|Texas Instruments Incorporated
|Low-Power, 2/8-Channel, 24-Bit Analog Front-End for Biopotential Measurements
| Marketing part#  Digital I/O Voltage Range   Package-type   #pins
|ADS1291IPBS   1.65V to 3.6 V   TQFP   32
|ADS1291IPBSR   1.65V to 3.6 V   TQFP   32
|ADS1291IRSMT   1.65V to 3.6 V   QFN   32
|ADS1291IRSMR   1.65V to 3.6 V   QFN   32
|ADS1292IPBS   1.65V to 3.6 V   TQFP   32
|ADS1292IPBSR   1.65V to 3.6 V   TQFP   32
|ADS1292RIPBS   1.65V to 3.6 V   TQFP   32
|ADS1292RIPBSR   1.65V to 3.6 V   TQFP   32
|ADS1292IRSMT   1.65V to 3.6 V   QFN   32
|ADS1292IRSMR   1.65V to 3.6 V   QFN   32
|ADS1292RIRSMT   1.65V to 3.6 V   QFN   32
|ADS1292RIRSMR   1.65V to 3.6 V   QFN   32
|ADS1294CZXGR   1.65V to 3.6 V   NFBGA   64
|ADS1294CZXGT   1.65V to 3.6 V   NFBGA   64
|ADS1294IPAG   1.65V to 3.6 V   PQFP   64
|ADS1294IPAGR   1.65V to 3.6 V   PQFP   64
|ADS1294RIZXGT   1.65V to 3.6 V   NFBGA   64
|ADS1294RIZXGR   1.65V to 3.6 V   NFBGA   64
|ADS1296CZXGR   1.65V to 3.6 V   NFBGA   64
|ADS1296CZXGT   1.65V to 3.6 V   NFBGA   64
|ADS1296IPAG   1.65V to 3.6 V   PQFP   64
|ADS1296IPAGR   1.65V to 3.6 V   PQFP   64
|ADS1296RIZXGT   1.65V to 3.6 V   NFBGA   64
|ADS1296RIZXGR   1.65V to 3.6 V   NFBGA   64
|ADS1298CZXGR   1.65V to 3.6 V   NFBGA   64
|ADS1298CZXGT   1.65V to 3.6 V   NFBGA   64
|ADS1298IPAG   1.65V to 3.6 V   PQFP   64
|ADS1298IPAGR   1.65V to 3.6 V   PQFP   64
|ADS1298RIZXGT   1.65V to 3.6 V   NFBGA   64
|ADS1298RIZXGR   1.65V to 3.6 V   NFBGA   64
|ADS1299CPAG   1.8V to 3.6 V   PQFP   64
|ADS1299CPAGR   1.8V to 3.6 V   PQFP   64
[IBIS Ver]   4.0
[File name]   ads129x.ibs
[File Rev]   1.0
[Date]   11/07/2011
[Source]   Texas Instruments Incorporated.
   Analog-eLab, HPA
   12500 TI Blvd
   Dallas, TX -75243
   For Support e-mail: elab_ibis@list.ti.com
[Notes]   Revision History:
   1.0: 01/24/2010 Initial Release
   2.0: 01/27/2010 Added ads1194/6/8 and ads1294/96
   3.0: 04/30/2010 Added marketing names for ads1294 and ads1296
   - Pin assignment based on product prelim data sheet
   ads1298.pdf
   - Initial version of the model
   - Initial Model generated from simulations in TISPICED
   - Model not matched to measurements
   - Ignore warnings related to c_comp, These are
   based on PVT variations as seen in simulations
   4.0: 11/02/2010
   - Removed references to ADS1192, ADS1196, and ADS1198 from file
   - Corrected C_comp values to true typ, min and max
   5.0: 11/18/2010
   - Added ADS1296R, ADS1294R, and ADS1294R products to this ibis
   file
   - Added ZXG R_pkg, L_pkg, and C_pkg values to the ADS1294, ADS1296,
   and ADS1298 prodcuts
   - Corrected all R_pkg, L_pkg, and C_pkg values to exclude GND and
   POWER pins from calculation
   6.0: 02/17/2011
   - Updated part numbers. The ending acronym RBZXGT is changed to RIZXGT
   and the ending acronym RBZXGR is changed to RIZXGR.
   6.1: 03/18/2011
   - Corrected part numbers to sure ADS1298R grades,
   6.2: 03/23/2011
   - Added ADS1299 products to this model.
   7.0: 04/05/2011
   - Added ADS1292 products in 32 pin TQFN package,
   8.0: 10/05/2011
   - Changed all GPIO buffers to DIO buffers. Both buffers are identical.
   - Added C_comp values that were simulated using a tank method. This
   method uses a 1nH inductor and a 1u ohm resistor.
   9.0  10/18/2011
   - Added 2.0 buffers with lagging _2 for ADS1291, ADS1292, and ADS1292R
   devices. 1.8 buffers with lagging _18 are buffers for ADS1294, ADS1296,
   and ADS1298.
   - Combined pullup data for DOUTRI_2, DIO_2, and CLK_2 is minor and
   verified with SPICE simulaton.
   10.0 11/07/2011
   - Changed voltage range for ADS1291, ADS1292, and ADS1292R. Lagging _2
   models still used with ADS1299.
   11.0 08/24/2012
   - 32 QFN package models added for ADS1291 and ADS1292
[Disclaimer]
 This product is designed as an aid for customers of Texas Instruments.
 No warranties, either expressed or implied, with respect to this third
 party software (if any) or with respect to its fitness for any
 particular purpose is claimed by Texas Instruments or the author. The
 software (if any) is provided solely on an "as is" basis. The entire
 risk as to its quality and performance is with the customer
[Copyright] (C) Copyright 2011 Texas Instruments Incorporated.
   All rights reserved.
|   ADS1299
[Component]   ads1299pag
[Manufacturer] TI
[Package]   |PAG (PQFP) - 64 pin
| variable   typ   min   max
R_pkg  0.007601   0.007601   0.007601
L_pkg  1.950031nH 1.950031nH 1.950031nH
C_pkg  0.403260pF 0.403260pF 0.403260pF
[Pin] signal_name   model_name   R_pin   L_pin   C_pin
1   IN8N   TERM   0.00802  2.18050nH  0.36893pF
2   IN8P   TERM   0.00796  2.08284nH  0.44422pF
3   IN7N   TERM   0.00774  2.00579nH  0.43874pF
4   IN7P   TERM   0.00761  1.96075nH  0.41947pF
5   IN6N   TERM   0.00767  1.93366nH  0.41193pF
6   IN6P   TERM   0.00745  1.86807nH  0.39172pF
7   IN5N   TERM   0.00723  1.80701nH  0.38069pF
8   IN5P   TERM   0.00717  1.80128nH  0.34665pF
9   IN4N   TERM   0.00717  1.80167nH  0.34655pF
10   IN4P   TERM   0.00723  1.80708nH  0.38064pF
11   IN3N   TERM   0.00746  1.86875nH  0.39156pF
12   IN3P   TERM   0.00767  1.93382nH  0.41197pF
13   IN2N   TERM   0.00762  1.96069nH  0.41976pF
14   IN2P   TERM   0.00774  2.00536nH  0.43931pF
15   IN1N   TERM   0.00796  2.08200nH  0.44472pF
16   IN1P   TERM   0.00802  2.18040nH  0.36892pF
17   TESTP_PACE_OUT1   TERM   0.00802  2.18050nH  0.36893pF
18   TESTP_PACE_OUT2   TERM   0.00796  2.08284nH  0.44422pF
19   AVDD   POWER   0.00774  2.00579nH  0.43874pF
20   AVSS   GND   0.00761  1.96075nH  0.41948pF
21   AVDD   POWER   0.00767  1.93365nH  0.41193pF
22   AVDD   POWER   0.00745  1.86807nH  0.39171pF
23   AVSS   GND   0.00723  1.80701nH  0.38069pF
24   VREFP   TERM   0.00717  1.80128nH  0.34665pF
25   VREFN   TERM   0.00717  1.80166nH  0.34656pF
26   VCAP4   TERM   0.00723  1.80707nH  0.38065pF
27   NC   NC   0.00746  1.86875nH  0.39156pF
28   VCAP1   TERM   0.00767  1.93381nH  0.41197pF
29   NC   NC   0.00762  1.96066nH  0.41979pF
30   VCAP2   TERM   0.00774  2.00511nH  0.43938pF
31   RESV1   DINPUT  0.00796  2.08195nH  0.44475pF
32   AVSS   GND   0.00802  2.18014nH  0.36899pF
33   DGND   GND   0.00802  2.18049nH  0.36893pF
34   DIN   DINPUT  0.00796  2.08283nH  0.44422pF
35   _PWDN   DINPUT  0.00774  2.00579nH  0.43874pF
36   _RESET   DINPUT  0.00761  1.96075nH  0.41947pF
37   CLK   CLK   0.00767  1.93366nH  0.41193pF
38   START   DINPUT  0.00745  1.86807nH  0.39172pF
39   _CS   DINPUT  0.00723  1.80701nH  0.38069pF
40   SCLK   DIO   0.00717  1.80128nH  0.34665pF
41   DAISY_IN   DIO   0.00717  1.80167nH  0.34655pF
42   GPIO1   DIO   0.00723  1.80708nH  0.38064pF
43   DOUT   DOUTRI  0.00746  1.86875nH  0.39156pF
44   GPIO2   DIO   0.00767  1.93382nH  0.41197pF
45   GPIO3   DIO   0.00762  1.96069nH  0.41976pF
46   GPIO4   DIO   0.00774  2.00536nH  0.43931pF
47   _DRDY   DOUTRI  0.00796  2.08200nH  0.44472pF
48   DVDD   POWER   0.00802  2.18040nH  0.36892pF
49   DGND   GND   0.00802  2.18051nH  0.36893pF
50   DVDD   POWER   0.00796  2.08284nH  0.44422pF
51   DGND   GND   0.00774  2.00579nH  0.43874pF
52   CLKSEL   DINPUT  0.00761  1.96073nH  0.41948pF
53   AVSS1   GND   0.00767  1.93366nH  0.41193pF
54   AVDD1   POWER   0.00745  1.86807nH  0.39171pF
55   VCAP3   TERM   0.00723  1.80701nH  0.38069pF
56   AVDD   POWER   0.00717  1.80128nH  0.34665pF
57   AVSS   GND   0.00717  1.80166nH  0.34656pF
58   AVSS   GND   0.00723  1.80707nH  0.38065pF
59   AVDD   POWER   0.00746  1.86875nH  0.39156pF
60   RLDREF   TERM   0.00767  1.93381nH  0.41197pF
61   RLDINV   TERM   0.00762  1.96066nH  0.41979pF
62   RLDIN   TERM   0.00774  2.00511nH  0.43938pF
63   RLDOUT   TERM   0.00796  2.08195nH  0.44475pF
64   WCT   TERM   0.00802  2.18014nH  0.36899pF
|   ADS1298
[Component]   ads1298zxg
[Manufacturer] TI
[Package]   |ZXG (PBGA) - 64 pin
| variable   typ   min   max
R_pkg  0.084959   0.084959   0.084959
L_pkg  1.726943nH 1.173300nH 2.802300nH
C_pkg  0.203317pF 0.155540pF 0.299270pF
[Pin] signal_name  model_name  R_pin  L_pin C_pin
1A   IN8P   TERM   0.080388   1.4891nH   0.16542pF
1B   IN7P   TERM   0.078742   1.4385nH   0.15797pF
1C   IN6P   TERM   0.077541   1.4231nH   0.16358pF
1D   IN5P   TERM   0.077252   1.4431nH   0.1602pF
1E   IN4P   TERM   0.076274   1.3909nH   0.16718pF
1F   IN3P   TERM   0.077401   1.4187nH   0.16692pF
1G   IN2P   TERM   0.077837   1.4526nH   0.16507pF
1H   IN1P   TERM   0.078364   1.4744nH   0.17666pF
2A   IN8N   TERM   0.078094   1.596nH   0.17296pF
2B   IN7N   TERM   0.077317   1.4768nH   0.18195pF
2C   IN6N   TERM   0.077292   1.453nH   0.17672pF
2D   IN5N   TERM   0.077416   1.4637nH   0.18795pF
2E   IN4N   TERM   0.076298   1.4016nH   0.17505pF
2F   IN3N   TERM   0.077508   1.4721nH   0.18998pF
2G   IN2N   TERM   0.077513   1.4687nH   0.18021pF
2H   IN1N   TERM   0.078587   1.5113nH   0.18073pF
3A   RLDIN   TERM   0.102240   2.3458nH   0.26608pF
3B   RLDOUT   TERM   0.086863   1.6155nH   0.20095pF
3C   RLDINV   TERM   0.098035   1.9627nH   0.23315pF
3D   WCT   TERM   0.078064   1.3941nH   0.17929pF
3E   TESTP_PACE_OUT1  TERM   0.114980   2.3577nH   0.25137pF
3F   TESTP_PACE_OUT2  TERM   0.101990   1.9882nH   0.23409pF
3G   VCAP4   TERM   0.091413   2.2569nH   0.21474pF
3H   VREFP   TERM   0.080602   1.5178nH   0.1901pF
4A   AVDD   POWER   0.044670   1.3107nH   0.45357pF
4B   AVDD   POWER   0.048649   1.5792nH   1.8442pF
4C   RLDREF   TERM   0.103750   1.931nH   0.22469pF
4D   AVSS   GND   0.014600   0.597nH   1.24pF
4E   RESV1   DINPUT   0.114160   2.8023nH   0.29927pF
4F   RESV2   TERM   0.085973   1.7256nH   0.21186pF
4G   RESV3   TERM   0.112330   2.1892nH   0.26167pF
4H   VREFN   TERM   0.071212   1.1733nH   0.16553pF
5A   AVSS   GND   0.015100   0.507nH   1.05pF
5B   AVSS   GND   0.014500   0.525nH   1.09pF
5C   AVSS   GND   0.014600   0.51nH   1.06pF
5D   AVSS   GND   0.015500   0.565nH   1.17pF
5E   GPIO4   DIO   0.106300   2.5339nH   0.28001pF
5F   GPIO1   DIO   0.103490   2.3545nH   0.28012pF
5G   _PWDN   DINPUT   0.097505   2.4515nH   0.26295pF
5H   VCAP1   TERM   0.079667   1.5368nH   0.19309pF
6A   AVDD   POWER   0.075279   1.207nH   0.57044pF
6B   AVDD   POWER   0.092725   2.1302nH   1.3472pF
6C   AVDD   POWER   0.084386   2.0005nH   1.1222pF
6D   _DRDY   DOUTRI   0.091680   2.019nH   0.23826pF
6E   GPIO3   DIO   0.092806   2.0233nH   0.22887pF
6F   DAISY_IN  DIO   0.088617   1.947nH   0.2188pF
6G   _RESET   DINPUT   0.086990   1.8608nH   0.22873pF
6H   VCAP2   TERM   0.071069   1.1744nH   0.15554pF
7A   AVDD1   POWER   0.077645   1.5948nH   0.30025pF
7B   VCAP3   TERM   0.051511   1.7265nH   0.2824pF
7C   DGND   GND   0.081013   1.9004nH   2.5639pF
7D   DGND   GND   0.054453   2.6508nH   1.2779pF
7E   GPIO2   DIO   0.079229   1.5455nH   0.20485pF
7F   _CS   DINPUT   0.076401   1.4359nH   0.20602pF
7G   START   DINPUT   0.078608   1.6115nH   0.19124pF
7H   DGND   GND   0.081108   1.8108nH   0.15779pF
8A   AVSS1   GND   0.044297   1.8219nH   0.26788pF
8B   CLKSEL   DINPUT   0.098048   2.1296nH   0.20021pF
8C   DVDD   POWER   0.073395   1.2676nH   0.87513pF
8D   DVDD   POWER   0.043758   1.9585nH   1.3668pF
8E   DOUT   DOUTRI   0.074125   1.4171nH   0.18957pF
8F   SCLK   DIO   0.073385   1.4896nH   0.17876pF
8G   CLK   CLK   0.073365   1.5643nH   0.15694pF
8H   DIN   DINPUT   0.084824   1.7114nH   0.1582pF
[Component]   ads1298pag
[Manufacturer] TI
[Package]   |PAG (PQFP) - 64 pin
| variable   typ   min   max
R_pkg  0.007601   0.007601   0.007601
L_pkg  1.950031nH 1.950031nH 1.950031nH
C_pkg  0.403260pF 0.403260pF 0.403260pF
[Pin] signal_name   model_name   R_pin   L_pin   C_pin
1   IN8N   TERM   0.00802  2.18050nH  0.36893pF
2   IN8P   TERM   0.00796  2.08284nH  0.44422pF
3   IN7N   TERM   0.00774  2.00579nH  0.43874pF
4   IN7P   TERM   0.00761  1.96075nH  0.41947pF
5   IN6N   TERM   0.00767  1.93366nH  0.41193pF
6   IN6P   TERM   0.00745  1.86807nH  0.39172pF
7   IN5N   TERM   0.00723  1.80701nH  0.38069pF
8   IN5P   TERM   0.00717  1.80128nH  0.34665pF
9   IN4N   TERM   0.00717  1.80167nH  0.34655pF
10   IN4P   TERM   0.00723  1.80708nH  0.38064pF
11   IN3N   TERM   0.00746  1.86875nH  0.39156pF
12   IN3P   TERM   0.00767  1.93382nH  0.41197pF
13   IN2N   TERM   0.00762  1.96069nH  0.41976pF
14   IN2P   TERM   0.00774  2.00536nH  0.43931pF
15   IN1N   TERM   0.00796  2.08200nH  0.44472pF
16   IN1P   TERM   0.00802  2.18040nH  0.36892pF
17   TESTP_PACE_OUT1   TERM   0.00802  2.18050nH  0.36893pF
18   TESTP_PACE_OUT2   TERM   0.00796  2.08284nH  0.44422pF
19   AVDD   POWER   0.00774  2.00579nH  0.43874pF
20   AVSS   GND   0.00761  1.96075nH  0.41948pF
21   AVDD   POWER   0.00767  1.93365nH  0.41193pF
22   AVDD   POWER   0.00745  1.86807nH  0.39171pF
23   AVSS   GND   0.00723  1.80701nH  0.38069pF
24   VREFP   TERM   0.00717  1.80128nH  0.34665pF
25   VREFN   TERM   0.00717  1.80166nH  0.34656pF
26   VCAP4   TERM   0.00723  1.80707nH  0.38065pF
27   NC   NC   0.00746  1.86875nH  0.39156pF
28   VCAP1   TERM   0.00767  1.93381nH  0.41197pF
29   NC   NC   0.00762  1.96066nH  0.41979pF
30   VCAP2   TERM   0.00774  2.00511nH  0.43938pF
31   RESV1   DINPUT  0.00796  2.08195nH  0.44475pF
32   AVSS   GND   0.00802  2.18014nH  0.36899pF
33   DGND   GND   0.00802  2.18049nH  0.36893pF
34   DIN   DINPUT  0.00796  2.08283nH  0.44422pF
35   _PWDN   DINPUT  0.00774  2.00579nH  0.43874pF
36   _RESET   DINPUT  0.00761  1.96075nH  0.41947pF
37   CLK   CLK   0.00767  1.93366nH  0.41193pF
38   START   DINPUT  0.00745  1.86807nH  0.39172pF
39   _CS   DINPUT  0.00723  1.80701nH  0.38069pF
40   SCLK   DIO   0.00717  1.80128nH  0.34665pF
41   DAISY_IN   DIO   0.00717  1.80167nH  0.34655pF
42   GPIO1   DIO   0.00723  1.80708nH  0.38064pF
43   DOUT   DOUTRI  0.00746  1.86875nH  0.39156pF
44   GPIO2   DIO   0.00767  1.93382nH  0.41197pF
45   GPIO3   DIO   0.00762  1.96069nH  0.41976pF
46   GPIO4   DIO   0.00774  2.00536nH  0.43931pF
47   _DRDY   DOUTRI  0.00796  2.08200nH  0.44472pF
48   DVDD   POWER   0.00802  2.18040nH  0.36892pF
49   DGND   GND   0.00802  2.18051nH  0.36893pF
50   DVDD   POWER   0.00796  2.08284nH  0.44422pF
51   DGND   GND   0.00774  2.00579nH  0.43874pF
52   CLKSEL   DINPUT  0.00761  1.96073nH  0.41948pF
53   AVSS1   GND   0.00767  1.93366nH  0.41193pF
54   AVDD1   POWER   0.00745  1.86807nH  0.39171pF
55   VCAP3   TERM   0.00723  1.80701nH  0.38069pF
56   AVDD   POWER   0.00717  1.80128nH  0.34665pF
57   AVSS   GND   0.00717  1.80166nH  0.34656pF
58   AVSS   GND   0.00723  1.80707nH  0.38065pF
59   AVDD   POWER   0.00746  1.86875nH  0.39156pF
60   RLDREF   TERM   0.00767  1.93381nH  0.41197pF
61   RLDINV   TERM   0.00762  1.96066nH  0.41979pF
62   RLDIN   TERM   0.00774  2.00511nH  0.43938pF
63   RLDOUT   TERM   0.00796  2.08195nH  0.44475pF
64   WCT   TERM   0.00802  2.18014nH  0.36899pF
|   ADS1296
[Component]   ads1296zxg
[Manufacturer] TI
[Package]   |ZXG (PBGA) - 64 pin
| variable   typ   min   max
R_pkg  0.084959   0.084959   0.084959
L_pkg  1.726943nH 1.173300nH 2.802300nH
C_pkg  0.203317pF 0.155540pF 0.299270pF
[Pin] signal_name  model_name  R_pin  L_pin C_pin
1A   NC   NC   0.080388   1.4891nH   0.16542pF
1B   NC   NC   0.078742   1.4385nH   0.15797pF
1C   IN6P   TERM   0.077541   1.4231nH   0.16358pF
1D   IN5P   TERM   0.077252   1.4431nH   0.1602pF
1E   IN4P   TERM   0.076274   1.3909nH   0.16718pF
1F   IN3P   TERM   0.077401   1.4187nH   0.16692pF
1G   IN2P   TERM   0.077837   1.4526nH   0.16507pF
1H   IN1P   TERM   0.078364   1.4744nH   0.17666pF
2A   NC   NC   0.078094   1.596nH   0.17296pF
2B   NC   NC   0.077317   1.4768nH   0.18195pF
2C   IN6N   TERM   0.077292   1.453nH   0.17672pF
2D   IN5N   TERM   0.077416   1.4637nH   0.18795pF
2E   IN4N   TERM   0.076298   1.4016nH   0.17505pF
2F   IN3N   TERM   0.077508   1.4721nH   0.18998pF
2G   IN2N   TERM   0.077513   1.4687nH   0.18021pF
2H   IN1N   TERM   0.078587   1.5113nH   0.18073pF
3A   RLDIN   TERM   0.102240   2.3458nH   0.26608pF
3B   RLDOUT   TERM   0.086863   1.6155nH   0.20095pF
3C   RLDINV   TERM   0.098035   1.9627nH   0.23315pF
3D   WCT   TERM   0.078064   1.3941nH   0.17929pF
3E   TESTP_PACE_OUT1  TERM   0.114980   2.3577nH   0.25137pF
3F   TESTP_PACE_OUT2  TERM   0.101990   1.9882nH   0.23409pF
3G   VCAP4   TERM   0.091413   2.2569nH   0.21474pF
3H   VREFP   TERM   0.080602   1.5178nH   0.1901pF
4A   AVDD   POWER   0.044670   1.3107nH   0.45357pF
4B   AVDD   POWER   0.048649   1.5792nH   1.8442pF
4C   RLDREF   TERM   0.103750   1.931nH   0.22469pF
4D   AVSS   GND   0.014600   0.597nH   1.24pF
4E   RESV1   DINPUT   0.114160   2.8023nH   0.29927pF
4F   RESV2   TERM   0.085973   1.7256nH   0.21186pF
4G   RESV3   TERM   0.112330   2.1892nH   0.26167pF
4H   VREFN   TERM   0.071212   1.1733nH   0.16553pF
5A   AVSS   GND   0.015100   0.507nH   1.05pF
5B   AVSS   GND   0.014500   0.525nH   1.09pF
5C   AVSS   GND   0.014600   0.51nH   1.06pF
5D   AVSS   GND   0.015500   0.565nH   1.17pF
5E   GPIO4   DIO   0.106300   2.5339nH   0.28001pF
5F   GPIO1   DIO   0.103490   2.3545nH   0.28012pF
5G   _PWDN   DINPUT   0.097505   2.4515nH   0.26295pF
5H   VCAP1   TERM   0.079667   1.5368nH   0.19309pF
6A   AVDD   POWER   0.075279   1.207nH   0.57044pF
6B   AVDD   POWER   0.092725   2.1302nH   1.3472pF
6C   AVDD   POWER   0.084386   2.0005nH   1.1222pF
6D   _DRDY   DOUTRI   0.091680   2.019nH   0.23826pF
6E   GPIO3   DIO   0.092806   2.0233nH   0.22887pF
6F   DAISY_IN  DIO   0.088617   1.947nH   0.2188pF
6G   _RESET   DINPUT   0.086990   1.8608nH   0.22873pF
6H   VCAP2   TERM   0.071069   1.1744nH   0.15554pF
7A   AVDD1   POWER   0.077645   1.5948nH   0.30025pF
7B   VCAP3   TERM   0.051511   1.7265nH   0.2824pF
7C   DGND   GND   0.081013   1.9004nH   2.5639pF
7D   DGND   GND   0.054453   2.6508nH   1.2779pF
7E   GPIO2   DIO   0.079229   1.5455nH   0.20485pF
7F   _CS   DINPUT   0.076401   1.4359nH   0.20602pF
7G   START   DINPUT   0.078608   1.6115nH   0.19124pF
7H   DGND   GND   0.081108   1.8108nH   0.15779pF
8A   AVSS1   GND   0.044297   1.8219nH   0.26788pF
8B   CLKSEL   DINPUT   0.098048   2.1296nH   0.20021pF
8C   DVDD   POWER   0.073395   1.2676nH   0.87513pF
8D   DVDD   POWER   0.043758   1.9585nH   1.3668pF
8E   DOUT   DOUTRI   0.074125   1.4171nH   0.18957pF
8F   SCLK   DIO   0.073385   1.4896nH   0.17876pF
8G   CLK   CLK   0.073365   1.5643nH   0.15694pF
8H   DIN   DINPUT   0.084824   1.7114nH   0.1582pF
[Component]   ads1296pag
[Manufacturer] TI
[Package]   |PAG (PQFP) - 64 pin
| variable   typ   min   max
R_pkg  0.007601   0.007601   0.007601
L_pkg  1.950031nH 1.950031nH 1.950031nH
C_pkg  0.403260pF 0.403260pF 0.403260pF
[Pin] signal_name   model_name   R_pin   L_pin   C_pin
1   NC   NC   0.00802  2.18050nH  0.36893pF
2   NC   NC   0.00796  2.08284nH  0.44422pF
3   NC   NC   0.00774  2.00579nH  0.43874pF
4   NC   NC   0.00761  1.96075nH  0.41947pF
5   IN6N   TERM   0.00767  1.93366nH  0.41193pF
6   IN6P   TERM   0.00745  1.86807nH  0.39172pF
7   IN5N   TERM   0.00723  1.80701nH  0.38069pF
8   IN5P   TERM   0.00717  1.80128nH  0.34665pF
9   IN4N   TERM   0.00717  1.80167nH  0.34655pF
10   IN4P   TERM   0.00723  1.80708nH  0.38064pF
11   IN3N   TERM   0.00746  1.86875nH  0.39156pF
12   IN3P   TERM   0.00767  1.93382nH  0.41197pF
13   IN2N   TERM   0.00762  1.96069nH  0.41976pF
14   IN2P   TERM   0.00774  2.00536nH  0.43931pF
15   IN1N   TERM   0.00796  2.08200nH  0.44472pF
16   IN1P   TERM   0.00802  2.18040nH  0.36892pF
17   TESTP_PACE_OUT1   TERM   0.00802  2.18050nH  0.36893pF
18   TESTP_PACE_OUT2   TERM   0.00796  2.08284nH  0.44422pF
19   AVDD   POWER   0.00774  2.00579nH  0.43874pF
20   AVSS   GND   0.00761  1.96075nH  0.41948pF
21   AVDD   POWER   0.00767  1.93365nH  0.41193pF
22   AVDD   POWER   0.00745  1.86807nH  0.39171pF
23   AVSS   GND   0.00723  1.80701nH  0.38069pF
24   VREFP   TERM   0.00717  1.80128nH  0.34665pF
25   VREFN   TERM   0.00717  1.80166nH  0.34656pF
26   VCAP4   TERM   0.00723  1.80707nH  0.38065pF
27   NC   NC   0.00746  1.86875nH  0.39156pF
28   VCAP1   TERM   0.00767  1.93381nH  0.41197pF
29   NC   NC   0.00762  1.96066nH  0.41979pF
30   VCAP2   TERM   0.00774  2.00511nH  0.43938pF
31   RESV1   DINPUT  0.00796  2.08195nH  0.44475pF
32   AVSS   GND   0.00802  2.18014nH  0.36899pF
33   DGND   GND   0.00802  2.18049nH  0.36893pF
34   DIN   DINPUT  0.00796  2.08283nH  0.44422pF
35   _PWDN   DINPUT  0.00774  2.00579nH  0.43874pF
36   _RESET   DINPUT  0.00761  1.96075nH  0.41947pF
37   CLK   CLK   0.00767  1.93366nH  0.41193pF
38   START   DINPUT  0.00745  1.86807nH  0.39172pF
39   _CS   DINPUT  0.00723  1.80701nH  0.38069pF
40   SCLK   DIO   0.00717  1.80128nH  0.34665pF
41   DAISY_IN   DIO   0.00717  1.80167nH  0.34655pF
42   GPIO1   DIO   0.00723  1.80708nH  0.38064pF
43   DOUT   DOUTRI  0.00746  1.86875nH  0.39156pF
44   GPIO2   DIO   0.00767  1.93382nH  0.41197pF
45   GPIO3   DIO   0.00762  1.96069nH  0.41976pF
46   GPIO4   DIO   0.00774  2.00536nH  0.43931pF
47   _DRDY   DOUTRI  0.00796  2.08200nH  0.44472pF
48   DVDD   POWER   0.00802  2.18040nH  0.36892pF
49   DGND   GND   0.00802  2.18051nH  0.36893pF
50   DVDD   POWER   0.00796  2.08284nH  0.44422pF
51   DGND   GND   0.00774  2.00579nH  0.43874pF
52   CLKSEL   DINPUT  0.00761  1.96073nH  0.41948pF
53   AVSS1   GND   0.00767  1.93366nH  0.41193pF
54   AVDD1   POWER   0.00745  1.86807nH  0.39171pF
55   VCAP3   TERM   0.00723  1.80701nH  0.38069pF
56   AVDD   POWER   0.00717  1.80128nH  0.34665pF
57   AVSS   GND   0.00717  1.80166nH  0.34656pF
58   AVSS   GND   0.00723  1.80707nH  0.38065pF
59   AVDD   POWER   0.00746  1.86875nH  0.39156pF
60   RLDREF   TERM   0.00767  1.93381nH  0.41197pF
61   RLDINV   TERM   0.00762  1.96066nH  0.41979pF
62   RLDIN   TERM   0.00774  2.00511nH  0.43938pF
63   RLDOUT   TERM   0.00796  2.08195nH  0.44475pF
64   WCT   TERM   0.00802  2.18014nH  0.36899pF
|   ADS1294
[Component]   ads1294zxg
[Manufacturer] TI
[Package]   |ZXG (PBGA) - 64 pin
| variable   typ   min   max
R_pkg  0.084959   0.084959   0.084959
L_pkg  1.726943nH 1.173300nH 2.802300nH
C_pkg  0.203317pF 0.155540pF 0.299270pF
[Pin] signal_name  model_name  R_pin  L_pin C_pin
1A   NC   NC   0.080388   1.4891nH   0.16542pF
1B   NC   NC   0.078742   1.4385nH   0.15797pF
1C   NC   NC   0.077541   1.4231nH   0.16358pF
1D   NC   NC   0.077252   1.4431nH   0.1602pF
1E   IN4P   TERM   0.076274   1.3909nH   0.16718pF
1F   IN3P   TERM   0.077401   1.4187nH   0.16692pF
1G   IN2P   TERM   0.077837   1.4526nH   0.16507pF
1H   IN1P   TERM   0.078364   1.4744nH   0.17666pF
2A   NC   NC   0.078094   1.596nH   0.17296pF
2B   NC   NC   0.077317   1.4768nH   0.18195pF
2C   NC   NC   0.077292   1.453nH   0.17672pF
2D   NC   NC   0.077416   1.4637nH   0.18795pF
2E   IN4N   TERM   0.076298   1.4016nH   0.17505pF
2F   IN3N   TERM   0.077508   1.4721nH   0.18998pF
2G   IN2N   TERM   0.077513   1.4687nH   0.18021pF
2H   IN1N   TERM   0.078587   1.5113nH   0.18073pF
3A   RLDIN   TERM   0.102240   2.3458nH   0.26608pF
3B   RLDOUT   TERM   0.086863   1.6155nH   0.20095pF
3C   RLDINV   TERM   0.098035   1.9627nH   0.23315pF
3D   WCT   TERM   0.078064   1.3941nH   0.17929pF
3E   TESTP_PACE_OUT1  TERM   0.114980   2.3577nH   0.25137pF
3F   TESTP_PACE_OUT2  TERM   0.101990   1.9882nH   0.23409pF
3G   VCAP4   TERM   0.091413   2.2569nH   0.21474pF
3H   VREFP   TERM   0.080602   1.5178nH   0.1901pF
4A   AVDD   POWER   0.044670   1.3107nH   0.45357pF
4B   AVDD   POWER   0.048649   1.5792nH   1.8442pF
4C   RLDREF   TERM   0.103750   1.931nH   0.22469pF
4D   AVSS   GND   0.014600   0.597nH   1.24pF
4E   RESV1   DINPUT   0.114160   2.8023nH   0.29927pF
4F   RESV2   TERM   0.085973   1.7256nH   0.21186pF
4G   RESV3   TERM   0.112330   2.1892nH   0.26167pF
4H   VREFN   TERM   0.071212   1.1733nH   0.16553pF
5A   AVSS   GND   0.015100   0.507nH   1.05pF
5B   AVSS   GND   0.014500   0.525nH   1.09pF
5C   AVSS   GND   0.014600   0.51nH   1.06pF
5D   AVSS   GND   0.015500   0.565nH   1.17pF
5E   GPIO4   DIO   0.106300   2.5339nH   0.28001pF
5F   GPIO1   DIO   0.103490   2.3545nH   0.28012pF
5G   _PWDN   DINPUT   0.097505   2.4515nH   0.26295pF
5H   VCAP1   TERM   0.079667   1.5368nH   0.19309pF
6A   AVDD   POWER   0.075279   1.207nH   0.57044pF
6B   AVDD   POWER   0.092725   2.1302nH   1.3472pF
6C   AVDD   POWER   0.084386   2.0005nH   1.1222pF
6D   _DRDY   DOUTRI   0.091680   2.019nH   0.23826pF
6E   GPIO3   DIO   0.092806   2.0233nH   0.22887pF
6F   DAISY_IN  DIO   0.088617   1.947nH   0.2188pF
6G   _RESET   DINPUT   0.086990   1.8608nH   0.22873pF
6H   VCAP2   TERM   0.071069   1.1744nH   0.15554pF
7A   AVDD1   POWER   0.077645   1.5948nH   0.30025pF
7B   VCAP3   TERM   0.051511   1.7265nH   0.2824pF
7C   DGND   GND   0.081013   1.9004nH   2.5639pF
7D   DGND   GND   0.054453   2.6508nH   1.2779pF
7E   GPIO2   DIO   0.079229   1.5455nH   0.20485pF
7F   _CS   DINPUT   0.076401   1.4359nH   0.20602pF
7G   START   DINPUT   0.078608   1.6115nH   0.19124pF
7H   DGND   GND   0.081108   1.8108nH   0.15779pF
8A   AVSS1   GND   0.044297   1.8219nH   0.26788pF
8B   CLKSEL   DINPUT   0.098048   2.1296nH   0.20021pF
8C   DVDD   POWER   0.073395   1.2676nH   0.87513pF
8D   DVDD   POWER   0.043758   1.9585nH   1.3668pF
8E   DOUT   DOUTRI   0.074125   1.4171nH   0.18957pF
8F   SCLK   DIO   0.073385   1.4896nH   0.17876pF
8G   CLK   CLK   0.073365   1.5643nH   0.15694pF
8H   DIN   DINPUT   0.084824   1.7114nH   0.1582pF
[Component]   ads1294pag
[Manufacturer] TI
[Package]   |PAG (PQFP) - 64 pin
| variable   typ   min   max
R_pkg  0.007601   0.007601   0.007601
L_pkg  1.950031nH 1.950031nH 1.950031nH
C_pkg  0.403260pF 0.403260pF 0.403260pF
[Pin] signal_name   model_name   R_pin   L_pin   C_pin
1   IN8N   NC   0.00802  2.18050nH  0.36893pF
2   IN8P   NC   0.00796  2.08284nH  0.44422pF
3   IN7N   NC   0.00774  2.00579nH  0.43874pF
4   IN7P   NC   0.00761  1.96075nH  0.41947pF
5   IN6N   NC   0.00767  1.93366nH  0.41193pF
6   IN6P   NC   0.00745  1.86807nH  0.39172pF
7   IN5N   NC   0.00723  1.80701nH  0.38069pF
8   IN5P   NC   0.00717  1.80128nH  0.34665pF
9   IN4N   TERM   0.00717  1.80167nH  0.34655pF
10   IN4P   TERM   0.00723  1.80708nH  0.38064pF
11   IN3N   TERM   0.00746  1.86875nH  0.39156pF
12   IN3P   TERM   0.00767  1.93382nH  0.41197pF
13   IN2N   TERM   0.00762  1.96069nH  0.41976pF
14   IN2P   TERM   0.00774  2.00536nH  0.43931pF
15   IN1N   TERM   0.00796  2.08200nH  0.44472pF
16   IN1P   TERM   0.00802  2.18040nH  0.36892pF
17   TESTP_PACE_OUT1   TERM   0.00802  2.18050nH  0.36893pF
18   TESTP_PACE_OUT2   TERM   0.00796  2.08284nH  0.44422pF
19   AVDD   POWER   0.00774  2.00579nH  0.43874pF
20   AVSS   GND   0.00761  1.96075nH  0.41948pF
21   AVDD   POWER   0.00767  1.93365nH  0.41193pF
22   AVDD   POWER   0.00745  1.86807nH  0.39171pF
23   AVSS   GND   0.00723  1.80701nH  0.38069pF
24   VREFP   TERM   0.00717  1.80128nH  0.34665pF
25   VREFN   TERM   0.00717  1.80166nH  0.34656pF
26   VCAP4   TERM   0.00723  1.80707nH  0.38065pF
27   NC   NC   0.00746  1.86875nH  0.39156pF
28   VCAP1   TERM   0.00767  1.93381nH  0.41197pF
29   NC   NC   0.00762  1.96066nH  0.41979pF
30   VCAP2   TERM   0.00774  2.00511nH  0.43938pF
31   RESV1   DINPUT  0.00796  2.08195nH  0.44475pF
32   AVSS   GND   0.00802  2.18014nH  0.36899pF
33   DGND   GND   0.00802  2.18049nH  0.36893pF
34   DIN   DINPUT  0.00796  2.08283nH  0.44422pF
35   _PWDN   DINPUT  0.00774  2.00579nH  0.43874pF
36   _RESET   DINPUT  0.00761  1.96075nH  0.41947pF
37   CLK   CLK   0.00767  1.93366nH  0.41193pF
38   START   DINPUT  0.00745  1.86807nH  0.39172pF
39   _CS   DINPUT  0.00723  1.80701nH  0.38069pF
40   SCLK   DIO   0.00717  1.80128nH  0.34665pF
41   DAISY_IN   DIO   0.00717  1.80167nH  0.34655pF
42   GPIO1   DIO   0.00723  1.80708nH  0.38064pF
43   DOUT   DOUTRI  0.00746  1.86875nH  0.39156pF
44   GPIO2   DIO   0.00767  1.93382nH  0.41197pF
45   GPIO3   DIO   0.00762  1.96069nH  0.41976pF
46   GPIO4   DIO   0.00774  2.00536nH  0.43931pF
47   _DRDY   DOUTRI  0.00796  2.08200nH  0.44472pF
48   DVDD   POWER   0.00802  2.18040nH  0.36892pF
49   DGND   GND   0.00802  2.18051nH  0.36893pF
50   DVDD   POWER   0.00796  2.08284nH  0.44422pF
51   DGND   GND   0.00774  2.00579nH  0.43874pF
52   CLKSEL   DINPUT  0.00761  1.96073nH  0.41948pF
53   AVSS1   GND   0.00767  1.93366nH  0.41193pF
54   AVDD1   POWER   0.00745  1.86807nH  0.39171pF
55   VCAP3   TERM   0.00723  1.80701nH  0.38069pF
56   AVDD   POWER   0.00717  1.80128nH  0.34665pF
57   AVSS   GND   0.00717  1.80166nH  0.34656pF
58   AVSS   GND   0.00723  1.80707nH  0.38065pF
59   AVDD   POWER   0.00746  1.86875nH  0.39156pF
60   RLDREF   TERM   0.00767  1.93381nH  0.41197pF
61   RLDINV   TERM   0.00762  1.96066nH  0.41979pF
62   RLDIN   TERM   0.00774  2.00511nH  0.43938pF
63   RLDOUT   TERM   0.00796  2.08195nH  0.44475pF
64   WCT   TERM   0.00802  2.18014nH  0.36899pF
|   ADS1292
[Component]   ads1292pbs
[Manufacturer] TI
[Package]   |PBS (TQFP) - 32 pin
| variable   typ   min   max
R_pkg   5.66263E-02   3.17700E-02   6.22300E-02
L_pkg   1.90859E+00nH 1.58036E+00nH 2.05660E+00nH
C_pkg   3.94649E-01pF 3.77910E-01pF 4.24640E-01pF
[Pin] signal_name   model_name   R_pin   L_pin   C_pin
1   PGA1N   TERM   0.06036  2.03101nH  0.37977pF
2   PGA1P   TERM   0.05911  1.95272nH  0.41005pF
3   IN1N   TERM   0.05831  1.88394nH  0.39201pF
4   IN1P   TERM   0.05810  1.84984nH  0.38129pF
5   IN2N   TERM   0.05810  1.85071nH  0.38135pF
6   IN2P   TERM   0.05832  1.88654nH  0.39223pF
7   PGA2N   TERM   0.05914  1.95753nH  0.41031pF
8   PGA2P   TERM   0.06041  2.03829nH  0.37970pF
9   VREFP   TERM   0.06011  2.03502nH  0.38025pF
10  VREFN   TERM   0.05849  1.94859nH  0.41037pF
11  VCAP1   TERM   0.05826  1.88956nH  0.39248pF
12  GPIO1/RCLK   DIO   0.03177  1.59232nH  0.41419pF
13  GPIO2/RCLK   DIO   0.03187  1.58036nH  0.41607pF
14  CLKSEL   DINPUT 0.05892  1.90189nH  0.39388pF
15  _PWDN/_RESET   DINPUT 0.05833  1.94540nH  0.41154pF
16  START   DINPUT 0.06005  2.03312nH  0.38068pF
17  CLK   CLK   0.06132  2.05652nH  0.38073pF
18  _CS   DINPUT 0.05940  1.96335nH  0.41136pF
19  DIN   DINPUT 0.05800  1.88100nH  0.39302pF
20  SCLK   DINPUT 0.05841  1.85614nH  0.38258pF
21  DOUT   DOUTRI 0.05918  1.86987nH  0.38231pF
22  _DRDY   DIO   0.05941  1.90531nH  0.39279pF
23  DVDD   POWER  0.06108  1.99071nH  0.41314pF
24  DGND   GND   0.06520  2.12375nH  0.38560pF
25  GPIO2/RCLK2   DIO   0.05982  2.02375nH  0.37791pF
26  GPIO1/RCLK1   DIO   0.05924  1.95629nH  0.40891pF
27  VCAP2   TERM   0.03343  1.67142nH  0.42464pF
28  RLDINV   TERM   0.06223  1.92683nH  0.38751pF
29  RLDIN/RLDREF   TERM   0.05963  1.87740nH  0.38482pF
30  RLDOUT   TERM   0.05832  1.88335nH  0.39358pF
31  RESP_MODP/IN3P TERM   0.05911  1.95300nH  0.41148pF
32  RESP_MODN/IN3N TERM   0.06164  2.05660nH  0.38167pF
|   ADS1292
[Component]   ads1292rsm
[Manufacturer] TI
[Package]   |RSM (QFN) - 32 pin
| variable   typ   min   max
R_pkg   0.0644   0.0330   0.0768
L_pkg   0.8006nH 0.5037nH 0.9598nH
C_pkg   0.1360pF 0.1213pF 0.1671pF
[Pin] signal_name   model_name   R_pin   L_pin   C_pin
1   PGA1N   TERM   0.06981   0.86398nH   0.12266pF
2   PGA1P   TERM   0.06734   0.82828nH   0.13736pF
3   IN1N   TERM   0.06549   0.80232nH   0.13536pF
4   IN1P   TERM   0.06467   0.7907nH   0.13341pF
5   IN2N   TERM   0.06467   0.7907nH   0.13342pF
6   IN2P   TERM   0.06549   0.80234nH   0.13537pF
7   PGA2N   TERM   0.06734   0.82831nH   0.1374pF
8   PGA2P   TERM   0.06982   0.86408nH   0.12324pF
9   VREFP   TERM   0.06941   0.85736nH   0.12314pF
10   VREFN   TERM   0.06537   0.79827nH   0.13606pF
11   VCAP1   TERM   0.06447   0.78457nH   0.1347pF
12   GPIO1/RCLK   DIO   0.03298   0.51461nH   0.1614pF
13   GPIO2/RCLK   DIO   0.03311   0.50367nH   0.16305pF
14   CLKSEL   DINPUT   0.06526   0.79658nH   0.13595pF
15   _PWDN/_RESET   DINPUT   0.06504   0.79185nH   0.13645pF
16   START   DINPUT   0.0693   0.85128nH   0.12337pF
17   CLK   CLK   0.07116   0.87727nH   0.1242pF
18   _CS   DINPUT   0.06777   0.82756nH   0.13844pF
19   DIN   DINPUT   0.06481   0.78556nH   0.13548pF
20   SCLK   DINPUT   0.06507   0.78889nH   0.13429pF
21   DOUT   DOUTRI   0.06646   0.80858nH   0.13514pF
22   _DRDY   DIO   0.0674   0.82218nH   0.13734pF
23   DVDD   POWER   0.07055   0.86775nH   0.14182pF
24   DGND   GND   0.07677   0.95983nH   0.13053pF
25   GPIO2/RCLK2   DIO   0.0689   0.84568nH   0.1213pF
26   GPIO1/RCLK1   DIO   0.06673   0.81477nH   0.13627pF
27   VCAP2   TERM   0.03588   0.58479nH   0.16713pF
28   RLDINV   TERM   0.07055   0.86802nH   0.14129pF
29   RLDIN/RLDREF   TERM   0.06633   0.80886nH   0.13681pF
30   RLDOUT   TERM   0.06454   0.78561nH   0.13566pF
31   RESP_MODP/IN3P   TERM   0.06653   0.81501nH   0.13796pF
32   RESP_MODN/IN3N   TERM   0.07165   0.89005nH   0.12572pF
|   ADS1291
[Component]   ads1291pbs
[Manufacturer] TI
[Package]   |PBS (TQFP) - 32 pin
| variable   typ   min   max
R_pkg   5.66263E-02   3.17700E-02   6.22300E-02
L_pkg   1.90859E+00nH 1.58036E+00nH 2.05660E+00nH
C_pkg   3.94649E-01pF 3.77910E-01pF 4.24640E-01pF
[Pin] signal_name   model_name   R_pin   L_pin   C_pin
1   PGA1N   TERM   0.06036  2.03101nH  0.37977pF
2   PGA1P   TERM   0.05911  1.95272nH  0.41005pF
3   IN1N   TERM   0.05831  1.88394nH  0.39201pF
4   IN1P   TERM   0.05810  1.84984nH  0.38129pF
5   IN2N   TERM   0.05810  1.85071nH  0.38135pF
6   IN2P   TERM   0.05832  1.88654nH  0.39223pF
7   PGA2N   TERM   0.05914  1.95753nH  0.41031pF
8   PGA2P   TERM   0.06041  2.03829nH  0.37970pF
9   VREFP   TERM   0.06011  2.03502nH  0.38025pF
10  VREFN   TERM   0.05849  1.94859nH  0.41037pF
11  VCAP1   TERM   0.05826  1.88956nH  0.39248pF
12  GPIO1/RCLK   DIO   0.03177  1.59232nH  0.41419pF
13  GPIO2/RCLK   DIO   0.03187  1.58036nH  0.41607pF
14  CLKSEL   DINPUT 0.05892  1.90189nH  0.39388pF
15  _PWDN/_RESET   DINPUT 0.05833  1.94540nH  0.41154pF
16  START   DINPUT 0.06005  2.03312nH  0.38068pF
17  CLK   CLK   0.06132  2.05652nH  0.38073pF
18  _CS   DINPUT 0.05940  1.96335nH  0.41136pF
19  DIN   DINPUT 0.05800  1.88100nH  0.39302pF
20  SCLK   DINPUT 0.05841  1.85614nH  0.38258pF
21  DOUT   DOUTRI 0.05918  1.86987nH  0.38231pF
22  _DRDY   DIO   0.05941  1.90531nH  0.39279pF
23  DVDD   POWER  0.06108  1.99071nH  0.41314pF
24  DGND   GND   0.06520  2.12375nH  0.38560pF
25  NC   TERM   0.05982  2.02375nH  0.37791pF
26  NC   TERM   0.05924  1.95629nH  0.40891pF
27  VCAP2   TERM   0.03343  1.67142nH  0.42464pF
28  RLDINV   TERM   0.06223  1.92683nH  0.38751pF
29  RLDIN/RLDREF   TERM   0.05963  1.87740nH  0.38482pF
30  RLDOUT   TERM   0.05832  1.88335nH  0.39358pF
31  RESP_MODP/IN3P TERM   0.05911  1.95300nH  0.41148pF
32  RESP_MODN/IN3N TERM   0.06164  2.05660nH  0.38167pF
|   ADS1291
[Component]   ads1291rsm
[Manufacturer] TI
[Package]   |RSM (QFN) - 32 pin
| variable   typ   min   max
R_pkg   0.0644   0.0330   0.0768
L_pkg   0.8006nH 0.5037nH 0.9598nH
C_pkg   0.1360pF 0.1213pF 0.1671pF
[Pin] signal_name   model_name   R_pin   L_pin   C_pin
1   PGA1N   TERM   0.06981   0.86398nH   0.12266pF
2   PGA1P   TERM   0.06734   0.82828nH   0.13736pF
3   IN1N   TERM   0.06549   0.80232nH   0.13536pF
4   IN1P   TERM   0.06467   0.7907nH   0.13341pF
5   IN2N   TERM   0.06467   0.7907nH   0.13342pF
6   IN2P   TERM   0.06549   0.80234nH   0.13537pF
7   PGA2N   TERM   0.06734   0.82831nH   0.1374pF
8   PGA2P   TERM   0.06982   0.86408nH   0.12324pF
9   VREFP   TERM   0.06941   0.85736nH   0.12314pF
10   VREFN   TERM   0.06537   0.79827nH   0.13606pF
11   VCAP1   TERM   0.06447   0.78457nH   0.1347pF
12   GPIO1/RCLK   DIO   0.03298   0.51461nH   0.1614pF
13   GPIO2/RCLK   DIO   0.03311   0.50367nH   0.16305pF
14   CLKSEL   DINPUT   0.06526   0.79658nH   0.13595pF
15   _PWDN/_RESET   DINPUT   0.06504   0.79185nH   0.13645pF
16   START   DINPUT   0.0693   0.85128nH   0.12337pF
17   CLK   CLK   0.07116   0.87727nH   0.1242pF
18   _CS   DINPUT   0.06777   0.82756nH   0.13844pF
19   DIN   DINPUT   0.06481   0.78556nH   0.13548pF
20   SCLK   DINPUT   0.06507   0.78889nH   0.13429pF
21   DOUT   DOUTRI   0.06646   0.80858nH   0.13514pF
22   _DRDY   DIO   0.0674   0.82218nH   0.13734pF
23   DVDD   POWER   0.07055   0.86775nH   0.14182pF
24   DGND   GND   0.07677   0.95983nH   0.13053pF
25   GPIO2/RCLK2   DIO   0.0689   0.84568nH   0.1213pF
26   GPIO1/RCLK1   DIO   0.06673   0.81477nH   0.13627pF
27   VCAP2   TERM   0.03588   0.58479nH   0.16713pF
28   RLDINV   TERM   0.07055   0.86802nH   0.14129pF
29   RLDIN/RLDREF   TERM   0.06633   0.80886nH   0.13681pF
30   RLDOUT   TERM   0.06454   0.78561nH   0.13566pF
31   RESP_MODP/IN3P   TERM   0.06653   0.81501nH   0.13796pF
32   RESP_MODN/IN3N   TERM   0.07165   0.89005nH   0.12572pF
[Model Selector]  DINPUT
DINPUT_18  1.8V digital input
DINPUT_2   2.0V digital input
DINPUT_33  3.3V digital input
|NOTES   Model DINPUT split into three Models DINPUT_18, DINPUT_2, and DINPUT_33
|   to accomodate voltage range of 1.65 V - 3.6V
|   DINPUT_18 operates in voltage range of 1.65 - 1.8 - 1.96
|   (specifically for ADS1294, ADS1296, and ADS1298 products)
|   DINPUT_2 operates in voltage range of 1.8 - 2.0 - 2.2
|   (specifically for ADS1291,ADS1292, ADS1292R, and ADS1299 products)
|   DINPUT_33 operates in voltage range of 3 - 3.3 - 3.6
|   (for all products)
|   The max pin frequency for Model DINPUT is 32 MHz.Also the
|   voltage range and frequency is referenced with datasheet.
[Model Selector]  CLK
CLK_18  1.8V digital I/O
CLK_2   2.0V digital I/O
CLK_33  3.3V digital I/O
|NOTES   Model CLK split into three Models CLK_18, CLK_2, and CLK_33
|   to accomodate voltage range of 1.65 V - 3.6V
|   CLK_18 operates in voltage range of 1.65 - 1.8 - 1.96
|   (specifically for ADS1294, ADS1296, and ADS1298 products)
|   CLK_2 operates in voltage range of 1.8 - 2.0 - 2.2
|   (specifically for ADS1291,ADS1292, ADS1292R, and ADS1299 products)
|   CLK_33 operates in voltage range of 3 - 3.3 - 3.6
|   (for all products)
|   The max pin frequency for Model CLK is 32 MHz.Also the
|   voltage range and frequency is referenced with datasheet.
[Model Selector] DIO
DIO_18  1.8V digital I/O
DIO_2   2.0V digital I/O
DIO_33  3.3V digital I/O
|NOTES   Model DIO split into three Models DIO_18, DIO_2, and DIO_33
|   to accomodate voltage range of 1.65 V - 3.6V
|   DIO_18 operates in voltage range of 1.65 - 1.8 - 1.96
|   (specifically for ADS1294, ADS1296, and ADS1298 products)
|   DIO_2 operates in voltage range of 1.8 - 2.0 - 2.2
|   (specifically for ADS1291,ADS1292, ADS1292R, and ADS1299 products)
|   DIO_33 operates in voltage range of 3 - 3.3 - 3.6
|   (for all products)
|   The max pin frequency for Model DIO is 32 MHz.Also the
|   voltage range and frequency is referenced with datasheet.
[Model Selector]  DOUTRI
DOUTRI_18  1.8V digital I/O
DOUTRI_2   2.0V digital I/O
DOUTRI_33  3.3V digital I/O
|NOTES   Model DOUTRI split into three Models DOUTRI_18, DOUTRI_2, and DOUTRI_33
|   to accomodate voltage range of 1.65 V - 3.6V
|   DOUTRI_18 operates in voltage range of 1.65 - 1.8 - 1.96
|   (specifically for ADS1294, ADS1296, and ADS1298 products)
|   DOUTRI_2 operates in voltage range of 1.8 - 2.0 - 2.2
|   (specifically for ADS1291,ADS1292, ADS1292R, and ADS1299 products)
|   DOUTRI_33 operates in voltage range of 3 - 3.3 - 3.6
|   (for all products)
|   The max pin frequency for Model DOUTRI is 32 MHz.Also the
|   voltage range and frequency is referenced with datasheet.
[Model Selector]  TERM
TERM_18  1.8V digital I/O
TERM_2   2.0V digital I/O
TERM_33  3.3V digital I/O
|   TERM Model
[Model] TERM_18
Model_type Terminator
|for ADS1291, ADS1292, ADS1294, ADS1296, and ADS1298 products
C_comp   1e-20   1e-20   1e-20
| variable   typ   min   max
[Voltage Range]   1.8V   1.65V   2V
[POWER Clamp Reference]  1.8V   1.65V   2V
[GND Clamp Reference]   0.0V   0.0V   0.0V
|Operating Temperature
[Temperature Range]   27   85   -40
|   TERM Model
[Model] TERM_2
Model_type Terminator
|for ADS1299 products
C_comp   1e-20   1e-20   1e-20
| variable   typ   min   max
[Voltage Range]   2.0V   1.8V   2.2V
[POWER Clamp Reference]  2.0V   1.8V   2.2V
[GND Clamp Reference]   0.0V   0.0V   0.0V
|Operating Temperature
[Temperature Range]   27   85   -40
|   TERM Model
[Model] TERM_33
Model_type Terminator
|for all products
C_comp   1e-20   1e-20   1e-20
| variable   typ   min   max
[Voltage Range]   3.3V   3.0V   3.6V
[POWER Clamp Reference]  3.3V   3.0V   3.6V
[GND Clamp Reference]   0.0V   0.0V   0.0V
|Operating Temperature
[Temperature Range]   27   85   -40
| Models and submodels in the file (15): DINPUT_18 (Input), DINPUT_2 (Input), DINPUT_33 (Input), CLK_18 (I/O), CLK_2 (I/O), CLK_33 (I/O), DIO_18 (I/O), DIO_2 (I/O), DIO_33 (I/O), DOUTRI_18 (I/O), DOUTRI_2 (I/O), DOUTRI_33 (I/O), TERM_18 (Terminator), TERM_2 (Terminator), TERM_33 (Terminator)
